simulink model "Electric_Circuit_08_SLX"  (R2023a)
settings: Solver=ode23s  StartTime=0.0  StopTime=10.0  MaxStep=0.001  RelTol=1e-3
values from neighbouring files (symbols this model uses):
  C_5 = 0.001*F    (= 0.001)    [Electric_Circuit_08_EQN.m]    (also in Electric_Circuit_08_SLX_m.m; Electric_Circuit_02_EQN.m; Electric_Circuit_02_SLX_m.m; Electric_Circuit_04_EQN.m)
  C_6 = 0.001*F    (= 0.001)    [Electric_Circuit_08_EQN.m]    (also in Electric_Circuit_08_SLX_m.m; Electric_Circuit_01_EQN.m; Electric_Circuit_01_SLX_m.m; Electric_Circuit_03_EQN.m)
  I_2_0 = 0*A    (= 0)    [Electric_Circuit_08_SLX_m.m]    (also in Electric_Circuit_02_SLX_m.m; Electric_Circuit_03_SLX_m.m; Electric_Circuit_06_SLX_m.m; Electric_Circuit_09_SLX_m.m)
  I_3_0 = 0*A    (= 0)    [Electric_Circuit_08_SLX_m.m]    (also in Electric_Circuit_10_SLX_m.m; Inductive_Circuit_2_SLX_m.m)
  I_8_0 = 0*A    (= 0)    [Electric_Circuit_08_SLX_m.m]    (also in Electric_Circuit_02_SLX_m.m; Electric_Circuit_05_SLX_m.m; Electric_Circuit_06_SLX_m.m; Electric_Circuit_07_SLX_m.m)
  L_2 = 0.002*H    (= 0.002)    [Electric_Circuit_08_EQN.m]    (also in Electric_Circuit_08_SLX_m.m; Electric_Circuit_02_EQN.m; Electric_Circuit_02_SLX_m.m; Electric_Circuit_03_EQN.m)
  L_3 = 0.002*H    (= 0.002)    [Electric_Circuit_08_EQN.m]    (also in Electric_Circuit_08_SLX_m.m; Electric_Circuit_10_EQN.m; Electric_Circuit_10_SLX_m.m; Hydraulic_Circuit_01_EQN.m = 10)
  R_4 = 100*Ohm    (= 100)    [Electric_Circuit_08_EQN.m]    (also in Electric_Circuit_08_SLX_m.m; BIG_EC_Simscape_EQN.m; BIG_EC_Simscape_SLX_m.m; Electric_Circuit_10_EQN.m)
  R_7 = 100*Ohm    (= 100)    [Electric_Circuit_08_EQN.m]    (also in Electric_Circuit_08_SLX_m.m; BIG_EC_Simscape_EQN.m; BIG_EC_Simscape_SLX_m.m; Electric_Circuit_03_EQN.m)
  Ts = Tfin/Nr_Ts_Points    (= 0.00014997)    [Electric_Circuit_08_SLX_m.m]    (also in BIG_EC_Simscape_SLX_m.m = 0.0003; Car_Dumper_SLX_m.m = 0.0022779; Electric_Circuit_01_SLX_m.m = 0.005; Electric_Circuit_02_SLX_m.m = 0.000480145)
  V_1_0 = 10*V    (= 10)    [Electric_Circuit_08_SLX_m.m]    (also in BIG_EC_Simscape_SLX_m.m; Electric_Circuit_02_SLX_m.m; Electric_Circuit_03_SLX_m.m; Electric_Circuit_04_SLX_m.m)
  V_5_0 = 0*V    (= 0)    [Electric_Circuit_08_SLX_m.m]    (also in Electric_Circuit_02_SLX_m.m; Electric_Circuit_04_SLX_m.m; Electric_Circuit_05_SLX_m.m)
  V_6_0 = 0*V    (= 0)    [Electric_Circuit_08_SLX_m.m]    (also in Electric_Circuit_01_SLX_m.m; Electric_Circuit_03_SLX_m.m; Electric_Circuit_06_SLX_m.m; Electric_Circuit_10_SLX_m.m)

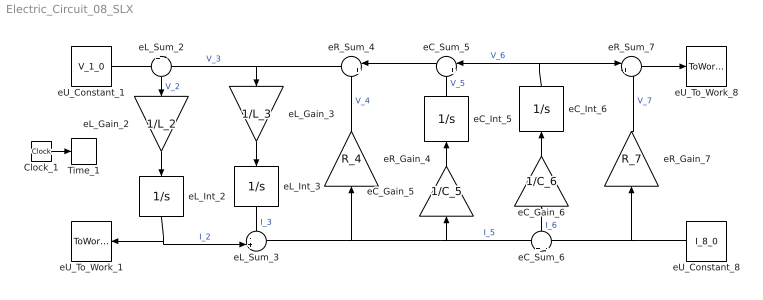
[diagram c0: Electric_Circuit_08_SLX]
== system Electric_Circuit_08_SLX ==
  Clock_1 : Clock
  Time_1 : ToWorkspace  VariableName=t  SaveFormat=Timeseries  SampleTime=Ts
  eC_Gain_5 : Gain  Gain=1/C_5  Multiplication=Matrix(K*u)
  eC_Gain_6 : Gain  Gain=1/C_6  Multiplication=Matrix(K*u)
  eC_Int_5 : Integrator  InitialCondition=V_5_0
  eC_Int_6 : Integrator  InitialCondition=V_6_0
  eC_Sum_5 : Sum  Inputs=|++
  eC_Sum_6 : Sum  Inputs=+|-
  eL_Gain_2 : Gain  Gain=1/L_2  Multiplication=Matrix(K*u)
  eL_Gain_3 : Gain  Gain=1/L_3  Multiplication=Matrix(K*u)
  eL_Int_2 : Integrator  InitialCondition=I_2_0
  eL_Int_3 : Integrator  InitialCondition=I_3_0
  eL_Sum_2 : Sum  Inputs=+|-
  eL_Sum_3 : Sum  Inputs=-+|
  eR_Gain_4 : Gain  Gain=R_4  Multiplication=Matrix(K*u)
  eR_Gain_7 : Gain  Gain=R_7  Multiplication=Matrix(K*u)
  eR_Sum_4 : Sum  Inputs=|++
  eR_Sum_7 : Sum  Inputs=|+-
  eU_Constant_1 : Constant  Value=V_1_0
  eU_Constant_8 : Constant  Value=I_8_0
  eU_To_Work_1 : ToWorkspace  VariableName=I_1_0  SaveFormat=Timeseries  SampleTime=Ts
  eU_To_Work_8 : ToWorkspace  VariableName=V_8_0  SaveFormat=Timeseries  SampleTime=Ts
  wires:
  eU_Constant_1/1 -> eL_Sum_2/1
  eR_Sum_4/1 -> eL_Sum_2/2, eL_Gain_3/1  "V_3"
  eL_Int_2/1 -> eU_To_Work_1/1, eL_Sum_3/2  "I_2"
  eL_Sum_2/1 -> eL_Gain_2/1  "V_2"
  eL_Gain_2/1 -> eL_Int_2/1
  eL_Sum_3/1 -> eR_Gain_4/1, eC_Gain_5/1, eC_Sum_6/1  "I_5"
  eL_Gain_3/1 -> eL_Int_3/1
  eL_Int_3/1 -> eL_Sum_3/1  "I_3"
  eC_Sum_5/1 -> eR_Sum_4/1
  eR_Gain_4/1 -> eR_Sum_4/2  "V_4"
  eC_Int_6/1 -> eC_Sum_5/1, eR_Sum_7/1  "V_6"
  eC_Gain_5/1 -> eC_Int_5/1
  eC_Int_5/1 -> eC_Sum_5/2  "V_5"
  eU_Constant_8/1 -> eC_Sum_6/2, eR_Gain_7/1
  eC_Sum_6/1 -> eC_Gain_6/1  "I_6"
  eC_Gain_6/1 -> eC_Int_6/1
  eR_Sum_7/1 -> eU_To_Work_8/1
  eR_Gain_7/1 -> eR_Sum_7/2  "V_7"
  Clock_1/1 -> Time_1/1
